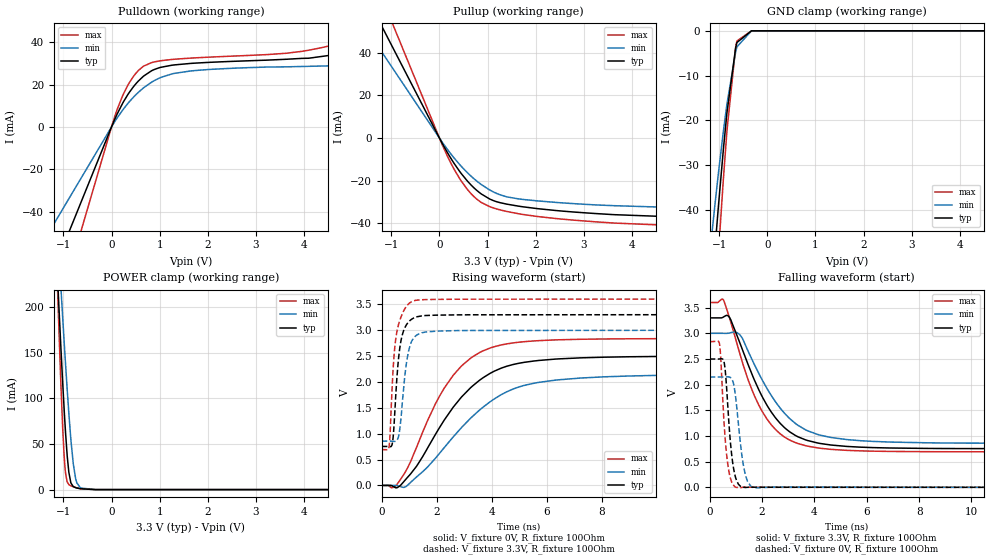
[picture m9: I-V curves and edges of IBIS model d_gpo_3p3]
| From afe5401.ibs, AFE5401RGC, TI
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|   d_gpo_3p3 Model
[Model]   d_gpo_3p3
Model_type   3-state
Polarity   Non-Inverting
Vmeas = 1.65
Vref = 0
Cref = 5pF
Rref = 100
|   typ   min   max
|   (nom PVT)   (fast PVT)   (slow PVT)
C_comp   1.561e-12   1.494e-12   1.659e-12
| Where nom  PVT is Nominal Process, 3.3V, 27C
|   Fast PVT is Strong Process,  3.6V, -40C
|   Slow PVT is Weak Process,   3V, 125C
[Voltage Range]   3.3   3   3.6
|Junction Temperature
[Temperature Range]   27   125   -40
[Pullup Reference]   3.3   3   3.6
[Pulldown Reference]   0   0   0
[Power Clamp Reference]   3.3   3   3.6
[GND Clamp Reference]   0   0   0
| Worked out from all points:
|   slope of the pulldown table from 0 to 0.495 V, typ, clamps not added: 24.7 ohm
|   slope of the pullup table from 0 to 0.495 V, typ, clamps not added: 27.8 ohm
|   POWER clamp passes 1 mA (typ) near -0.65 V on its own axis
|   falling waveform, V_fixture 3.3V, R_fixture 100Ohm: 20-80 % time 1.5ns typ, 1.64ns min, 1.35ns max; typ from 3.3 V to 0.752 V
|   rising waveform, V_fixture 0V, R_fixture 100Ohm: 20-80 % time 2.06ns typ, 2.44ns min, 1.7ns max; typ from 0 V to 2.5 V
|   rising waveform, V_fixture 3.3V, R_fixture 100Ohm: 20-80 % time 239ps typ, 268ps min, 244ps max; typ from 0.753 V to 3.3 V
|   falling waveform, V_fixture 0V, R_fixture 100Ohm: 20-80 % time 236ps typ, 288ps min, 213ps max; typ from 2.5 V to 0 V
[Pulldown]
|   Voltage   I(typ)   I(min)   I(max)
-3.3V     -185.1mA   -126.1mA   -255.8mA
-3mV      -168.3uA   -114.7uA   -232.5uA
231.6mV   11.2mA     7.956mA    14.74mA
366mV     16.2mA     11.79mA    20.74mA
559.2mV   21.7mA     16.37mA    26.67mA
831mV     26.51mA    21.11mA    30.36mA
1.261V    29.17mA    25.08mA    31.9mA
2.043V    30.53mA    27.17mA    32.99mA
4.102V    32.46mA    28.63mA    36.27mA
4.501V    33.71mA    28.84mA    38.15mA
5.833V    37.87mA    29.53mA    39.04mA
6.6V      40.26mA    29.92mA    52mA
[GND Clamp]
|   Voltage   I(typ)   I(min)   I(max)
-3.3V     -1.237A    -1.056A    -1.383A
-1.185V   -62.02mA   -48.47mA   -79.23mA
-1.09V    -48.68mA   -38.74mA   -62.09mA
-1.016V   -38.95mA   -31.63mA   -49.47mA
-914.1mV  -26.39mA   -22.38mA   -33mA
-840mV    -18.26mA   -16.29mA   -22.27mA
-660mV    -3.853mA   -4.762mA   -3.675mA
-632.4mV  -2.604mA   -3.574mA   -2.256mA
-330mV    -1.092uA   -13.07uA   -101.3nA
6.6V      0A         0A         0A
[Pullup]
|   Voltage   I(typ)   I(min)   I(max)
-3.3V     144.2mA    111mA      181.3mA
-3mV      131.1uA    100.9uA    164.8uA
260.7mV   -10.34mA   -8.102mA   -12.74mA
462mV     -16.88mA   -13.44mA   -20.42mA
724.8mV   -23.49mA   -19.2mA    -27.59mA
867.9mV   -26.16mA   -21.75mA   -30.15mA
1.046V    -28.58mA   -24.34mA   -32.15mA
1.398V    -30.95mA   -27.54mA   -34.39mA
1.647V    -31.91mA   -28.52mA   -35.47mA
2.835V    -34.73mA   -30.79mA   -38.55mA
5.098V    -36.9mA    -32.42mA   -41.35mA
6.6V      -36.9mA    -32.42mA   -41.35mA
[POWER Clamp]
|   Voltage   I(typ)   I(min)   I(max)
-3.3V     2.973A     2.513A     4.173A
-1.115V   224.2mA    279.7mA    208.8mA
-1.089V   194.8mA    255.2mA    168mA
-1.053V   155.8mA    222.2mA    115.5mA
-1.018V   119.2mA    190.5mA    69.8mA
-984mV    86.76mA    161.1mA    35.87mA
-956.4mV  62.6mA     137.8mA    18.2mA
-921mV    36.52mA    109mA      8.361mA
-841.5mV  6.984mA    52.62mA    4.074mA
-747mV    2.117mA    12.15mA    2.312mA
-645mV    931.7uA    1.77mA     936.9uA
6.6V      0A         0A         0A
[Ramp]
R_load = 100
|   typ   min   max
dV/dt_r   1.49945/2.05152e-09   1.28704/2.42774e-09   1.70286/1.69266e-09
dV/dt_f   1.52851/1.49582e-09   1.28663/1.63652e-09   1.7447/1.34967e-09
[Falling Waveform]
V_fixture = 3.3V
V_fixture_min = 3V
V_fixture_max = 3.6V
R_fixture = 100Ohm
|   Time   V(typ)   V(min)   V(max)
0s        3.3V       3V         3.6V
525ps     3.316V     3V         3.651V
755ps     3.314V     3.005V     3.303V
1.14ns    2.831V     2.978V     2.626V
1.645ns   2.168V     2.459V     1.861V
2.045ns   1.73V      2.056V     1.446V
2.695ns   1.246V     1.543V     1.042V
3.295ns   1.005V     1.237V     868.1mV
5.75ns    783.1mV    909.1mV    710.7mV
14.99ns   752.5mV    855.6mV    692.2mV
[Rising Waveform]
V_fixture = 0V
V_fixture_min = 0V
V_fixture_max = 0V
R_fixture = 100Ohm
|   Time   V(typ)   V(min)   V(max)
0s        1.34nV     67.89nV    678.2pV
445ps     -26.1mV    945.9uV    -35.44mV
880ps     121.7mV    -21.95mV   282.4mV
1.67ns    726.8mV    358.6mV    1.258V
2.275ns   1.266V     733mV      1.884V
2.92ns    1.72V      1.13V      2.319V
3.92ns    2.16V      1.609V     2.652V
5.005ns   2.362V     1.906V     2.769V
6.41ns    2.445V     2.04V      2.814V
14.99ns   2.499V     2.145V     2.838V
[Rising Waveform]
V_fixture = 3.3V
V_fixture_min = 3V
V_fixture_max = 3.6V
R_fixture = 100Ohm
|   Time   V(typ)   V(min)   V(max)
0s        753.3mV    855.6mV    693.3mV
270ps     750.9mV    856.1mV    757.5mV
410ps     911.2mV    853.4mV    2.215V
490ps     1.557V     851.8mV    2.748V
605ps     2.422V     934.1mV    3.098V
720ps     2.849V     1.418V     3.282V
910ps     3.115V     2.411V     3.47V
1.15ns    3.232V     2.842V     3.567V
2.75ns    3.296V     2.992V     3.598V
14.99ns   3.3V       3V         3.6V
[Falling Waveform]
V_fixture = 0V
V_fixture_min = 0V
V_fixture_max = 0V
R_fixture = 100Ohm
|   Time   V(typ)   V(min)   V(max)
0s        2.499V     2.148V     2.837V
375ps     2.5V       2.148V     2.794V
430ps     2.504V     2.148V     2.465V
550ps     2.439V     2.148V     1.258V
745ps     1.186V     2.15V      284.3mV
875ps     497.9mV    2.078V     65.35mV
1ns       175.1mV    1.723V     1.594mV
1.305ns   1.54mV     382.3mV    1.706mV
1.64ns    2.875mV    245.2uV    3.185mV
14.99ns   51.14nV    2.026uV    -148.8nV
